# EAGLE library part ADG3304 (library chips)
Bidirectional level translation; 1.15 V to 5.5 V; Low quiescent current <5 uA; No direction pin
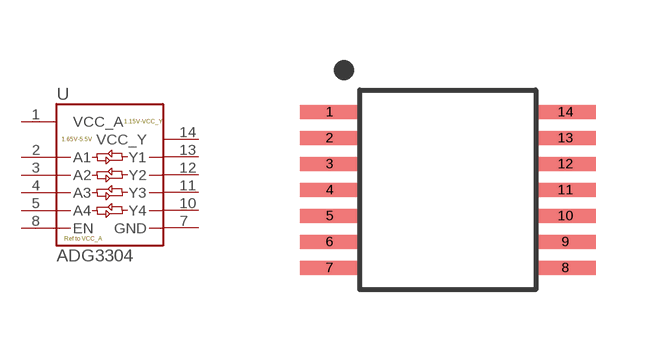
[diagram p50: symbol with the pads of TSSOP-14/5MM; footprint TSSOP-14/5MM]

Designator prefix U

## ADG3304 (DIGIKEY: ADG3304BRUZ-ND)  [TSSOP-14/5MM]
1  VCC_A
2  A1
3  A2
4  A3
5  A4
7  GND
8  EN
10  Y4
11  Y3
12  Y2
13  Y1
14  VCC_Y

## Footprint TSSOP-14/5MM (pad centres in mm)
smd 1.5 x 0.35: 1 -2.95,1.95; 2 -2.95,1.3; 3 -2.95,0.65; 4 -2.95,0; 5 -2.95,-0.65; 6 -2.95,-1.3; 7 -2.95,-1.95; 8 2.95,-1.95; 9 2.95,-1.3; 10 2.95,-0.65; 11 2.95,0; 12 2.95,0.65; 13 2.95,1.3; 14 2.95,1.95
